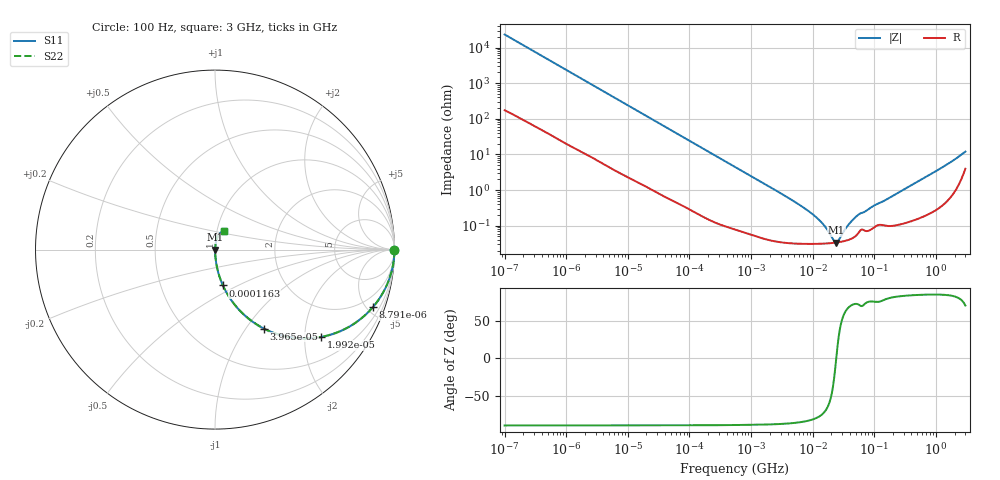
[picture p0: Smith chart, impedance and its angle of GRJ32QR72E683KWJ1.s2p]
!Murata Part Number: GRJ32QR72E683KWJ1
!These Parameters are Measured in Series Mode Connection
!Data Generated on Jun 19, 2026
!  o--ll--o
!Port1  Port2
!  o------o
!Operation Temp=25[degC], DC Bias Voltage=0[V]
!Freq. Start=100[Hz] Stop=3[GHz] 401[Steps]
# Hz S RI R 50
!Freq.(Hz) S11(Real) S11(Imag) S21(Real) S21(Imag) S12(Real) S12(Imag) S22(Real) S22(Imag)
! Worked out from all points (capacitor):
!   401 points, 100 Hz to 3 GHz, reference 50 ohm
!   read as one part in series: C = 68.1 nF near 109 Hz
!   lowest |Z| = 33.6 mohm at 24.18 MHz (marker M1)
!   series resonance near 24.06 MHz, so ESL is about 640 pH
!   S11 on the Smith chart (normalised r, x): 100 Hz: open; 8.791 kHz: 1.05, -5.45; 19.92 kHz: 1.02, -2.42; 39.66 kHz: 1.01, -1.22; 116.3 kHz: 1.00, -0.42; 3 GHz: 1.08, +0.23
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100  0.9999 -0.00428  5.02e-05 0.00428  5.02e-05 0.00428  0.9999 -0.00428
1788  0.9937 -0.0749  0.0063 0.0749  0.0063 0.0749  0.9937 -0.0749
4610  0.9624 -0.1857  0.0376 0.1857  0.0376 0.1857  0.9624 -0.1857
8791  0.8788 -0.3216  0.1212 0.3216  0.1212 0.3216  0.8788 -0.3216
12951  0.7721 -0.4145  0.2279 0.4145  0.2279 0.4145  0.7721 -0.4145
19917  0.5925 -0.4863  0.4075 0.4863  0.4075 0.4863  0.5925 -0.4863
31977  0.3643 -0.476  0.6357 0.476  0.6357 0.476  0.3643 -0.476
39655  0.273 -0.4402  0.727 0.4402  0.727 0.4402  0.273 -0.4402
66468  0.1203 -0.3196  0.8797 0.3196  0.8797 0.3196  0.1203 -0.3196
116311  0.0442 -0.1996  0.9558 0.1996  0.9558 0.1996  0.0442 -0.1996
547723  0.00278 -0.0447  0.9972 0.0447  0.9972 0.0447  0.00278 -0.0447
3966702  0.000361 -0.0061  0.9996 0.0061  0.9996 0.0061  0.000361 -0.0061
9794414  0.000312 -0.00212  0.9997 0.00212  0.9997 0.00212  0.000312 -0.00212
1.442825e7  0.000313 -0.00111  0.9997 0.00111  0.9997 0.00111  0.000313 -0.00111
2.12544e7  0.000327 -0.000258  0.9997 0.000258  0.9997 0.000258  0.000327 -0.000258
2.418395e7  0.000336 1.08e-05  0.9997 -1.08e-05  0.9997 -1.08e-05  0.000336 1.08e-05
2.635803e7  0.000343 0.00019  0.9997 -0.00019  0.9997 -0.00019  0.000343 0.00019
3.71925e7  0.000394 0.000936  0.9996 -0.000936  0.9996 -0.000936  0.000394 0.000936
5.248048e7  0.000565 0.00181  0.9994 -0.00181  0.9994 -0.00181  0.000565 0.00181
1.751444e8  0.00101 0.00595  0.999 -0.00595  0.999 -0.00595  0.00101 0.00595
9.797344e8  0.00377 0.033  0.9962 -0.033  0.9962 -0.033  0.00377 0.033
3e9  0.0494 0.1037  0.9506 -0.1037  0.9506 -0.1037  0.0494 0.1037
